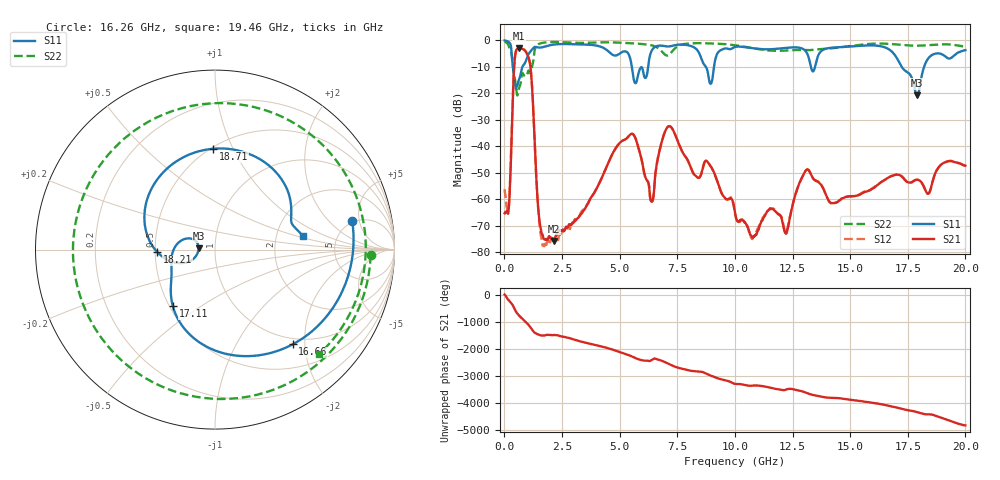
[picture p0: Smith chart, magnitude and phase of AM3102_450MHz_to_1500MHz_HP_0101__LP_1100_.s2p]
!Agilent Technologies,E8364B,MY43040894,A.07.50.67
!Agilent E8364B: A.07.50.67
!Date: Thursday, January 11, 2018 05:43:01
!Correction: S11(Full 2 Port(1,2))
!S21(Full 2 Port(1,2))
!S12(Full 2 Port(1,2))
!S22(Full 2 Port(1,2))
!S2P File: Measurements: S11, S21, S12, S22:
# Hz S  dB  R 50
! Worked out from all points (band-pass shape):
!   1601 points, 10 MHz to 20 GHz, reference 50 ohm
!   highest |S21| = -2.96 dB at 634.7 MHz (marker M1); lowest = -75.6 dB at 2.146 GHz (marker M2)
!   |S21| within 3 dB of the highest: 464.2 MHz to 1.023 GHz (558.9 MHz wide, 75.2 % of centre)
!   lowest |S11| = -20.8 dB at 17.9 GHz (marker M3), VSWR 1.20, Z = 41.6 + j0.605 ohm
!   |S11| at or under -10 dB: 366 MHz to 782.7 MHz (416.7 MHz wide, 72.5 % of centre); 5.529 GHz to 6.237 GHz (708.3 MHz wide, 12 % of centre); 17.24 GHz to 18.21 GHz (971.5 MHz wide, 5.48 % of centre)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
!   |S22| runs from -20.8 to -0.5 dB; largest |S21 - S12| = 0.0021
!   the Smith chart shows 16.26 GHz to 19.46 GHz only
!   S11 on the Smith chart (normalised r, x): 16.26 GHz: 4.78, +3.95; 16.66 GHz: 0.89, -1.76; 17.11 GHz: 0.52, -0.39; 18.21 GHz: 0.51, -0.02; 18.71 GHz: 0.51, +0.84; 19.46 GHz: 2.84, +0.56
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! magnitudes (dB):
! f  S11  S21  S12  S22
! 10 MHz  -0.1  -65.2  -56.2  -0.5
! 184.9 MHz  -0.6  -64.0  -63.4  -2.1
! 447.3 MHz  -15.7  -7.4  -7.4  -14.1
! 634.7 MHz  -14.8  -3.0  -3.0  -18.1
! 1.122 GHz  -4.3  -9.4  -9.4  -12.2
! 1.609 GHz  -2.7  -72.4  -74.4  -1.1
! 2.146 GHz  -1.6  -75.6  -75.9  -0.6
! 3.346 GHz  -1.6  -65.3  -64.6  -1.0
! 5.445 GHz  -6.5  -35.6  -35.6  -1.1
! 6.682 GHz  -2.1  -43.5  -43.5  -3.0
! 10.01 GHz  -2.5  -65.0  -64.9  -1.9
! 12.22 GHz  -2.8  -72.9  -72.4  -3.9
! 13.34 GHz  -11.3  -51.3  -51.2  -3.6
! 16.26 GHz  -2.1  -54.0  -54.0  -1.2
! 16.66 GHz  -3.3  -51.7  -51.7  -1.3
! 16.68 GHz  -3.4  -51.7  -51.7  -1.3
! 17.11 GHz  -8.1  -50.7  -50.6  -1.7
! 17.9 GHz  -20.8  -52.6  -52.6  -2.0
! 18.21 GHz  -9.9  -55.5  -55.4  -1.9
! 18.71 GHz  -5.0  -49.7  -49.8  -1.6
! 19.46 GHz  -6.1  -45.7  -45.7  -1.7
! 20 GHz  -3.7  -47.3  -47.3  -2.4
